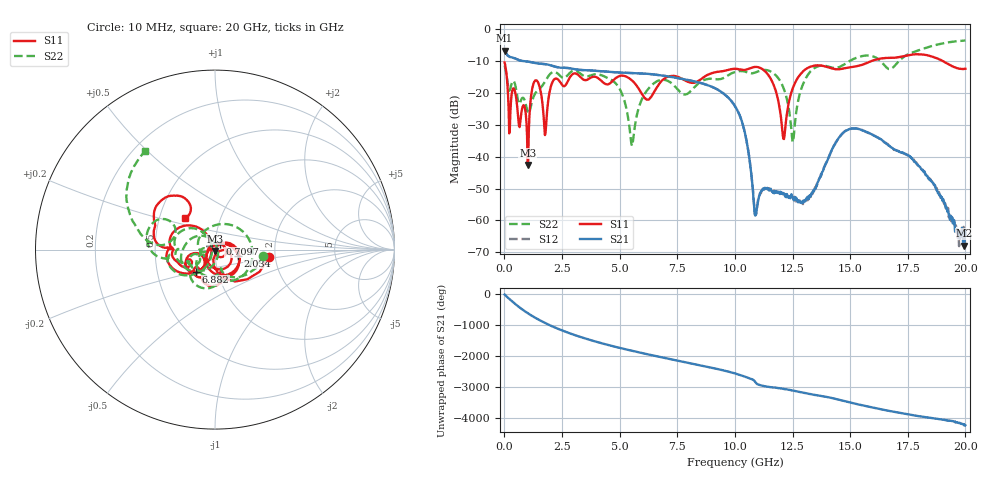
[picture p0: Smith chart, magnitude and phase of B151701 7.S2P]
!  2-Port S-parameters saved by WinCal
! VAR MeasName=S-Parameters (CALIBRATED_DATA) read from VNA (N5244A)
! VAR MeasDate=2015-12-24 19:08:55
! VAR NAME=B151701 7
! VAR FILENAME=B151701 7.S2P
! VAR DATE=2015-12-24 19:08:55
! VAR PHYS_PORTS=1,3
# Hz S DB R 50
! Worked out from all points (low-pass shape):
!   801 points, 10 MHz to 20 GHz, reference 50 ohm
!   highest |S21| = -6.65 dB at 10 MHz (marker M1); lowest = -67.9 dB at 19.95 GHz (marker M2)
!   |S21| within 3 dB of the highest: start of sweep to 637.1 MHz
!   lowest |S11| = -42.6 dB at 1.01 GHz (marker M3), VSWR 1.02, Z = 50.2 - j0.73 ohm
!   |S11| at or under -10 dB: start of sweep to 15.9 GHz; 19.04 GHz to end of sweep
!   |S22| runs from -36.6 to -3.5 dB; largest |S21 - S12| = 0.001
!   S11 on the Smith chart (normalised r, x): 10 MHz: 1.85, -0.17; 709.6 MHz: 1.05, +0.07; 2.034 GHz: 1.29, -0.09; 6.882 GHz: 0.79, -0.20; 20 GHz: 0.68, +0.25
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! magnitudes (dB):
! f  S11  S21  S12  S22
! 10 MHz  -10.4  -6.7  -6.7  -11.3
! 209.9 MHz  -32.6  -8.5  -8.5  -19.2
! 709.6 MHz  -27.8  -9.8  -9.8  -22.4
! 1.01 GHz  -42.6  -10.1  -10.1  -25.9
! 1.309 GHz  -16.3  -10.5  -10.5  -20.5
! 1.759 GHz  -33.2  -10.9  -10.9  -16.4
! 2.034 GHz  -17.5  -11.3  -11.3  -13.7
! 3.358 GHz  -15.3  -12.7  -12.7  -14.2
! 4.883 GHz  -15.0  -13.5  -13.5  -17.4
! 5.532 GHz  -16.0  -13.7  -13.7  -36.6
! 6.682 GHz  -17.5  -14.3  -14.3  -16.1
! 6.882 GHz  -15.8  -14.5  -14.5  -15.8
! 10.01 GHz  -12.4  -24.1  -24.1  -13.4
! 10.9 GHz  -11.8  -58.3  -58.3  -13.5
! 11.63 GHz  -16.6  -50.9  -50.8  -13.5
! 12.13 GHz  -34.4  -51.6  -51.8  -18.8
! 12.53 GHz  -18.1  -52.8  -52.8  -35.3
! 13.35 GHz  -11.5  -51.3  -51.3  -12.7
! 14.8 GHz  -12.1  -31.9  -31.8  -10.7
! 16.68 GHz  -8.9  -36.5  -36.4  -12.4
! 19.95 GHz  -12.4  -67.9  -62.5  -3.5
! 20 GHz  -12.3  -64.3  -63.4  -3.5
